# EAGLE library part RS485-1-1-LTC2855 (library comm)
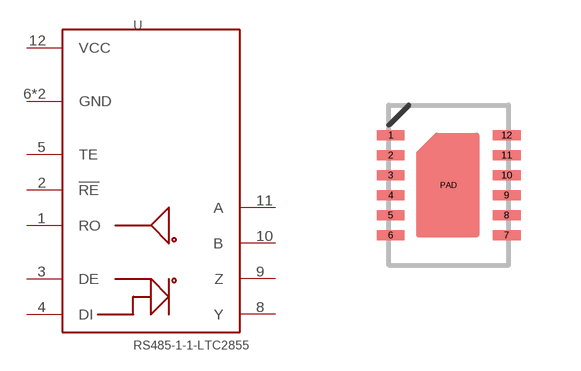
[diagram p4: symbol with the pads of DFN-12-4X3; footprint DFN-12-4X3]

Designator prefix U

## RS485-1-1-LTC2855  [DFN-12-4X3]
1  RO
2  !RE!
3  DE
4  DI
5  TE
6  GND
8  Y
9  Z
10  B
11  A
12  VCC
PAD  GND

## Footprint DFN-12-4X3 (pad centres in mm)
smd 0.7 x 0.25: 1 -1.45,1.25; 2 -1.45,0.75; 3 -1.45,0.25; 4 -1.45,-0.25; 5 -1.45,-0.75; 6 -1.45,-1.25; 7 1.45,-1.25; 8 1.45,-0.75; 9 1.45,-0.25; 10 1.45,0.25; 11 1.45,0.75; 12 1.45,1.25
smd 0.2 x 0.2: PAD 0,0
